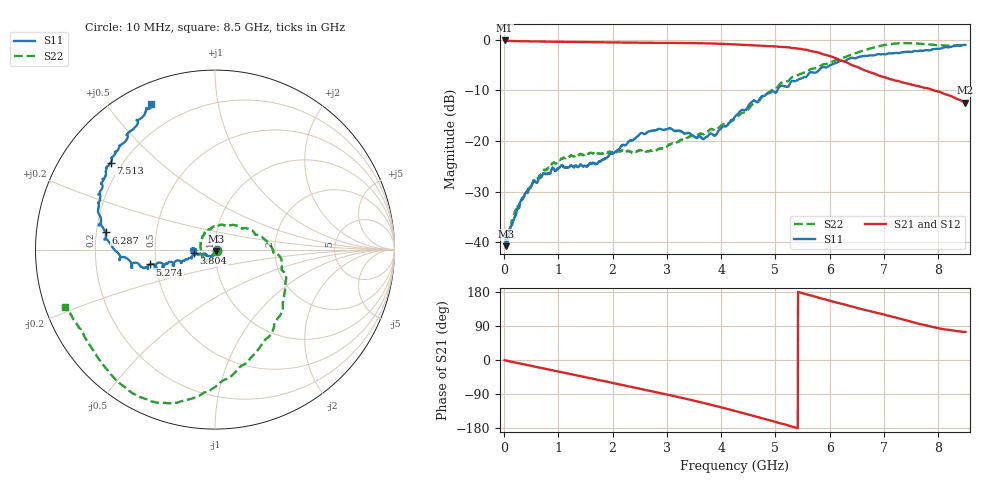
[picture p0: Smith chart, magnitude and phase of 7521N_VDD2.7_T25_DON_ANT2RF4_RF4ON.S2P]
!Agilent Technologies,E5071C,MY46417908,A.11.23
!Date: Thu Jul 30 15:13:59 2020
!Data & Calibration Information:
!Freq	S11:SOLT2(ON)	S21:SOLT2(ON)	S12:SOLT2(ON)	S22:SOLT2(ON)
!PortZ  Port1:50+j0  Port2:50+j0
!Above PortZ is port z conversion or system Z0 setting when saving the data.
!When reading, reference impedance value at option line is always used.
# Hz S dB R 50
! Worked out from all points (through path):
!   1601 points, 10 MHz to 8.5 GHz, reference 50 ohm
!   highest |S21| = -0.17 dB at 10 MHz (marker M1); lowest = -12.4 dB at 8.5 GHz (marker M2)
!   group delay of S21, straight-line fit = 97.5 ps
!   lowest |S11| = -40.8 dB at 36.53 MHz (marker M3), VSWR 1.02, Z = 50.5 - j0.748 ohm
!   |S11| at or under -10 dB: start of sweep to 5.036 GHz
!   |S22| runs from -40.4 to -0.7 dB; largest |S21 - S12| = 0.015
!   S11 on the Smith chart (normalised r, x): 10 MHz: 1.02, -0.00; 3.804 GHz: 0.79, -0.03; 5.274 GHz: 0.46, -0.09; 6.287 GHz: 0.24, +0.07; 7.513 GHz: 0.16, +0.35; 8.5 GHz: 0.09, +0.65
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1e7  -38.47 -11.5  -0.17 -0.6  -0.17 -0.6  -39.39 -31.0
3.653125e7  -40.78 -54.1  -0.22 -1.5  -0.23 -1.5  -40.36 -51.6
7.3675e7  -39.43 -67.7  -0.25 -2.6  -0.25 -2.6  -39.41 -70.2
2.169438e8  -34.71 -98.4  -0.30 -7.0  -0.30 -6.9  -33.72 -90.7
5.40625e8  -28.08 -116.3  -0.37 -16.7  -0.37 -16.6  -27.98 -106.0
9.067562e8  -25.39 -126.6  -0.43 -27.6  -0.43 -27.6  -24.29 -114.9
1.426769e9  -24.83 -145.6  -0.49 -43.1  -0.49 -43.1  -22.67 -124.5
1.723919e9  -24.42 -157.7  -0.52 -52.1  -0.52 -52.1  -22.48 -124.4
2.1325e9  -21.45 -164.7  -0.57 -64.6  -0.57 -64.7  -22.03 -137.0
2.509244e9  -18.51 -169.9  -0.61 -76.1  -0.61 -76.2  -21.79 -161.5
2.843538e9  -17.64 -176.4  -0.65 -86.3  -0.65 -86.5  -21.63 167.6
3.671312e9  -19.67 -176.3  -0.73 -113.2  -0.73 -113.5  -18.62 101.5
3.803969e9  -18.55 -170.4  -0.77 -117.9  -0.77 -118.1  -17.71 92.4
4.255e9  -15.20 -161.6  -0.96 -134.6  -0.95 -134.8  -15.60 55.6
4.753788e9  -11.17 -163.7  -1.23 -153.8  -1.20 -154.0  -11.40 15.5
5.2738e9  -8.55 -167.2  -1.59 -174.5  -1.56 -174.5  -7.75 -18.6
5.671769e9  -6.46 -167.6  -2.30 169.8  -2.28 169.6  -5.75 -45.4
6.287294e9  -4.19 171.1  -4.37 145.9  -4.38 145.4  -3.45 -78.6
6.738325e9  -3.10 158.4  -6.43 129.3  -6.38 130.2  -1.76 -95.9
7.088538e9  -2.70 150.0  -7.73 116.7  -7.62 118.5  -0.96 -107.2
7.513038e9  -2.41 140.2  -8.87 100.6  -8.84 102.7  -0.72 -121.7
8.5e9  -1.05 113.9  -12.43 74.0  -12.48 73.7  -0.96 -159.1
